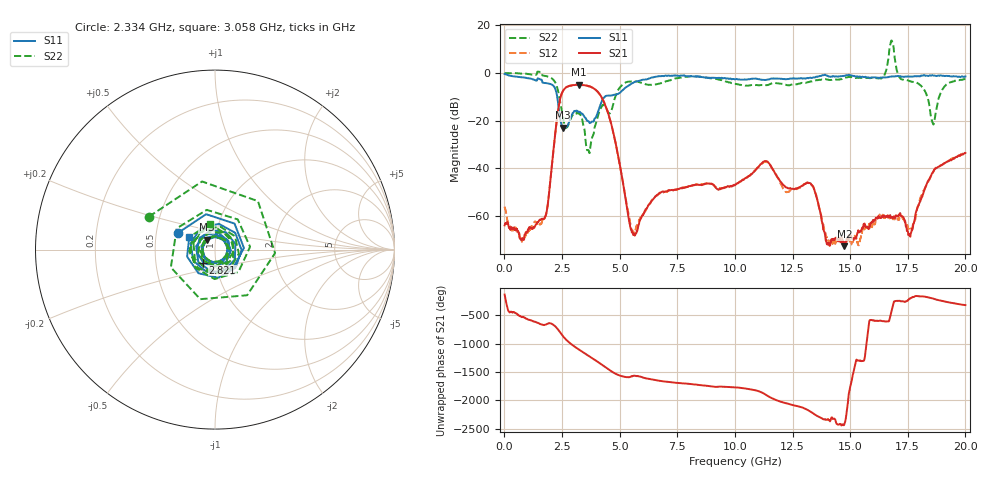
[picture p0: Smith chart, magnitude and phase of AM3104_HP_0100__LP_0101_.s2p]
!Created with skrf (http://scikit-rf.org).
# Hz S RI R 50.0
!freq ReS11 ImS11 ReS21 ImS21 ReS12 ImS12 ReS22 ImS22
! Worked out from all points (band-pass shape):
!   1601 points, 10 MHz to 20 GHz, reference 50 ohm
!   highest |S21| = -4.91 dB at 3.233 GHz (marker M1); lowest = -72.6 dB at 14.75 GHz (marker M2)
!   |S21| within 3 dB of the highest: 2.519 GHz to 4.054 GHz (1.535 GHz wide, 46.7 % of centre)
!   lowest |S11| = -22.9 dB at 2.534 GHz (marker M3), VSWR 1.15, Z = 45.4 + j5.06 ohm
!   |S11| at or under -10 dB: 2.293 GHz to 4.351 GHz (2.058 GHz wide, 62 % of centre)
!   |S22| runs from -33.6 to 13.6 dB; largest |S21 - S12| = 0.031
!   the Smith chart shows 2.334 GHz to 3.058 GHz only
!   S11 on the Smith chart (normalised r, x): 2.334 GHz: 0.65, +0.12; 2.821 GHz: 0.87, -0.13; 3.058 GHz: 0.74, +0.11
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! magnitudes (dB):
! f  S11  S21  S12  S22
! 10 MHz  -0.4  -63.8  -56.0  0.0
! 759.6 MHz  -1.8  -69.7  -70.7  -0.3
! 1.697 GHz  -4.2  -61.3  -60.9  -1.1
! 2.334 GHz  -12.9  -15.4  -15.4  -7.7
! 2.534 GHz  -22.9  -7.6  -7.7  -18.5
! 2.821 GHz  -20.2  -5.4  -5.4  -20.5
! 3.058 GHz  -15.9  -5.0  -5.0  -16.8
! 3.233 GHz  -16.4  -4.9  -5.0  -17.0
! 3.346 GHz  -16.9  -5.0  -5.1  -18.3
! 3.646 GHz  -20.2  -5.5  -5.6  -32.3
! 4.458 GHz  -9.5  -15.5  -15.5  -15.6
! 5.582 GHz  -4.1  -67.5  -66.6  -3.5
! 6.682 GHz  -1.4  -50.8  -50.8  -4.6
! 10.01 GHz  -2.7  -47.0  -46.9  -4.6
! 11.33 GHz  -2.9  -37.0  -37.3  -5.1
! 13.34 GHz  -2.1  -47.0  -47.1  -3.5
! 14.03 GHz  -1.3  -71.9  -69.3  -2.8
! 14.75 GHz  -1.2  -72.6  -71.5  -2.2
! 16.68 GHz  -1.6  -60.6  -60.2  7.2
! 17.61 GHz  -1.5  -68.6  -65.1  -3.4
! 18.59 GHz  -1.0  -41.7  -41.7  -21.1
! 20 GHz  -1.5  -33.5  -32.9  -2.5
